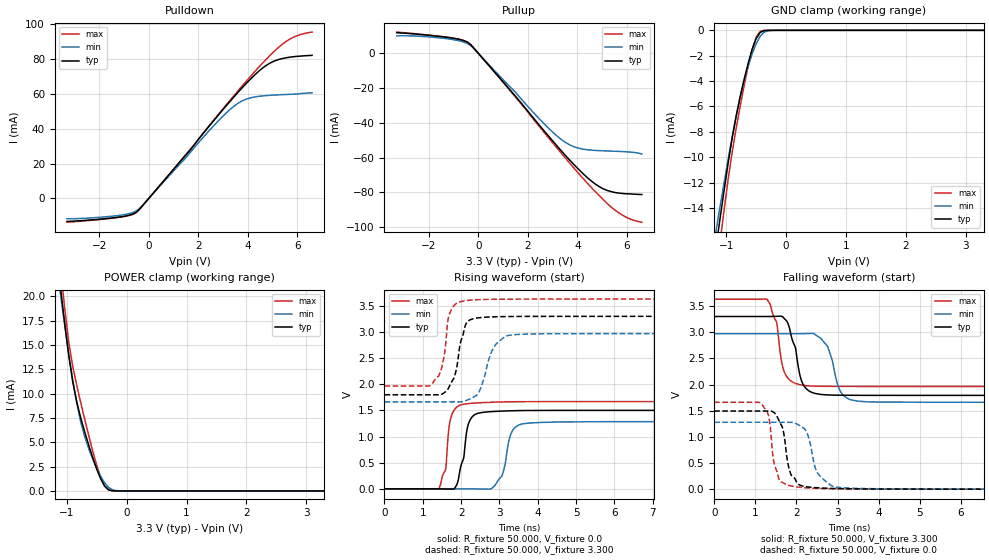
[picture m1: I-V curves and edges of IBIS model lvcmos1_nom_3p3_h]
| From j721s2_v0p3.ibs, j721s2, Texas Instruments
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|   nom_3p3_h
[Model]   lvcmos1_nom_3p3_h
Model_type I/O
Polarity   Non-Inverting
Enable   Active-High
Vinl = 0
Vinh = 0.8
Vmeas = 1.65
Vref = 3.3
Cref = 2pF
Rref = 100000
|   typ   min   max
C_comp   1.381pF   1.346pF   1.415pF
[Voltage Range]   3.3   2.97   3.63
[Temperature Range]   27   150   -40
[Pullup Reference]   3.3   2.97   3.63
[Pulldown Reference]   0   0   0
[Power Clamp Reference]   3.3   2.97   3.63
[GND Clamp Reference]   0   0   0
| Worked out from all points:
|   slope of the pulldown table from 0 to 0.495 V, typ, clamps not added: 60.2 ohm
|   slope of the pullup table from 0 to 0.495 V, typ, clamps not added: 61.1 ohm
|   GND clamp passes 1 mA (typ) near -0.53 V on its own axis
|   POWER clamp passes 1 mA (typ) near -0.41 V on its own axis
|   rising waveform, R_fixture 50.000, V_fixture 0.0: 20-80 % time 218ps typ, 220ps min, 151ps max; typ from 0 V to 1.5 V
|   rising waveform, R_fixture 50.000, V_fixture 3.300: 20-80 % time 269ps typ, 345ps min, 190ps max; typ from 1.8 V to 3.3 V
|   falling waveform, R_fixture 50.000, V_fixture 3.300: 20-80 % time 261ps typ, 271ps min, 232ps max; typ from 3.3 V to 1.79 V
|   falling waveform, R_fixture 50.000, V_fixture 0.0: 20-80 % time 207ps typ, 286ps min, 187ps max; typ from 1.49 V to 0 V
[Pulldown]
|Voltage   I(typ)   I(min)   I(max)
-3.3V     -13.19mA   -11.65mA   -13.61mA
-1.2V     -10.68mA   -9.718mA   -10.79mA
-500mV    -7.841mA   -7.111mA   -8.037mA
1.6V      26.5mA     25.04mA    26.88mA
2.7V      45.88mA    42.84mA    46.25mA
3.6V      60.77mA    54.51mA    61.61mA
4V        66.85mA    57.24mA    68.23mA
4.4V      72.38mA    58.47mA    74.56mA
5V        78.35mA    59.25mA    83.42mA
5.4V      80.25mA    59.54mA    88.46mA
5.8V      81.2mA     59.76mA    92.13mA
6.6V      82.08mA    60.57mA    95.42mA
[Pullup]
|Voltage   I(typ)   I(min)   I(max)
-3.3V     11.92mA    10.14mA    12.3mA
-1.4V     9.544mA    8.72mA     9.61mA
-800mV    8.191mA    7.383mA    8.222mA
-400mV    6.072mA    5.341mA    6.191mA
1V        -16.41mA   -15.13mA   -16.61mA
2.6V      -43.64mA   -39.7mA    -44.49mA
3.5V      -58.45mA   -51.06mA   -59.98mA
4.1V      -67.43mA   -54.72mA   -69.93mA
4.6V      -73.85mA   -55.7mA    -77.7mA
5V        -77.61mA   -56.03mA   -83.57mA
5.8V      -80.54mA   -56.46mA   -92.91mA
6.6V      -81.21mA   -57.9mA    -97.13mA
[GND_clamp]
|Voltage   I(typ)   I(min)   I(max)
-3.3V     -113.8mA   -82.24mA   -159mA
-1.167V   -17.01mA   -15.72mA   -19.19mA
-1.1V     -14.77mA   -13.85mA   -16.61mA
-1.033V   -12.58mA   -11.98mA   -14.09mA
-900mV    -8.5mA     -8.41mA    -9.615mA
-767mV    -5.246mA   -5.264mA   -6.001mA
-567mV    -1.506mA   -1.867mA   -1.524mA
-500mV    -657.8uA   -1.063mA   -541.1uA
-433mV    -173.4uA   -477.3uA   -85.64uA
-367mV    -24.15uA   -152.9uA   -5.315uA
-233mV    -388.3nA   -8.514uA   -220.5nA
3.3V      0A         0A         0A
[POWER_clamp]
|Voltage   I(typ)   I(min)   I(max)
-3.3V     168.5mA    143.2mA    197.8mA
-1.1V     20.63mA    20.01mA    22.61mA
-1.033V   17.13mA    16.96mA    18.69mA
-967mV    13.91mA    14.07mA    15.29mA
-900mV    11.2mA     11.4mA     12.78mA
-767mV    7.499mA    7.076mA    9.066mA
-633mV    4.696mA    4.33mA     5.68mA
-500mV    2.241mA    2.328mA    2.647mA
-367mV    494.4uA    820uA      496.9uA
-300mV    111.5uA    353.4uA    89.53uA
-100mV    169.5nA    4.704uA    108.2nA
3.3V      0A         0A         0A
[Ramp]
| variable   typ   min   max
dV/dt_r   0.900/0.218n   0.770/0.219n   1.001/0.150n
dV/dt_f   0.904/0.262n   0.784/0.270n   1.000/0.233n
R_load = 50.000
[Rising Waveform]
R_fixture= 50.000
V_fixture= 0.0
V_fixture_min= 0.0
V_fixture_max= 0.0
|time   V(typ)   V(min)   V(max)
0s        1.816uV    20.2uV     2.658uV
1.419ns   -469.7uV   95.09uV    3.247mV
1.599ns   -2.406mV   -141.4uV   386.3mV
1.741ns   -4.316mV   41.22uV    1.382V
2.02ns    497.5mV    -528.2uV   1.611V
2.318ns   1.399V     -1.888mV   1.639V
2.882ns   1.481V     63.94mV    1.658V
3.318ns   1.493V     1.081V     1.666V
3.588ns   1.497V     1.24V      1.667V
10ns      1.5V       1.284V     1.668V
[Rising Waveform]
R_fixture= 50.000
V_fixture= 3.300
V_fixture_min= 2.970
V_fixture_max= 3.630
|time   V(typ)   V(min)   V(max)
0s        1.799V     1.664V     1.967V
1.242ns   1.799V     1.664V     2.01V
1.472ns   1.803V     1.664V     2.261V
1.666ns   1.92V      1.664V     3.271V
1.806ns   2.108V     1.664V     3.499V
2.026ns   2.889V     1.666V     3.587V
2.445ns   3.27V      1.824V     3.619V
2.83ns    3.289V     2.678V     3.626V
3.25ns    3.296V     2.937V     3.628V
10ns      3.3V       2.97V      3.63V
[Falling Waveform]
R_fixture= 50.000
V_fixture= 3.300
V_fixture_min= 2.970
V_fixture_max= 3.630
|time   V(typ)   V(min)   V(max)
0s        3.3V       2.97V      3.63V
1.289ns   3.3V       2.97V      3.629V
1.521ns   3.304V     2.97V      3.176V
1.641ns   3.305V     2.97V      2.424V
1.771ns   3.205V     2.97V      2.145V
2.091ns   2.155V     2.972V     1.996V
2.735ns   1.803V     2.751V     1.966V
3.038ns   1.796V     1.918V     1.964V
3.336ns   1.794V     1.705V     1.964V
10ns      1.793V     1.663V     1.963V
[Falling Waveform]
R_fixture= 50.000
V_fixture= 0.0
V_fixture_min= 0.0
V_fixture_max= 0.0
|time   V(typ)   V(min)   V(max)
0s        1.493V     1.279V     1.661V
1.153ns   1.493V     1.279V     1.629V
1.317ns   1.493V     1.279V     1.413V
1.447ns   1.468V     1.279V     528.9mV
1.651ns   1.194V     1.279V     131.2mV
1.877ns   263.8mV    1.278V     61.02mV
2.249ns   45.86mV    1.089V     24.66mV
2.51ns    26.83mV    310.9mV    14.73mV
2.966ns   11.75mV    38.26mV    7.19mV
10ns      60.26uV    129.6uV    36.56uV
